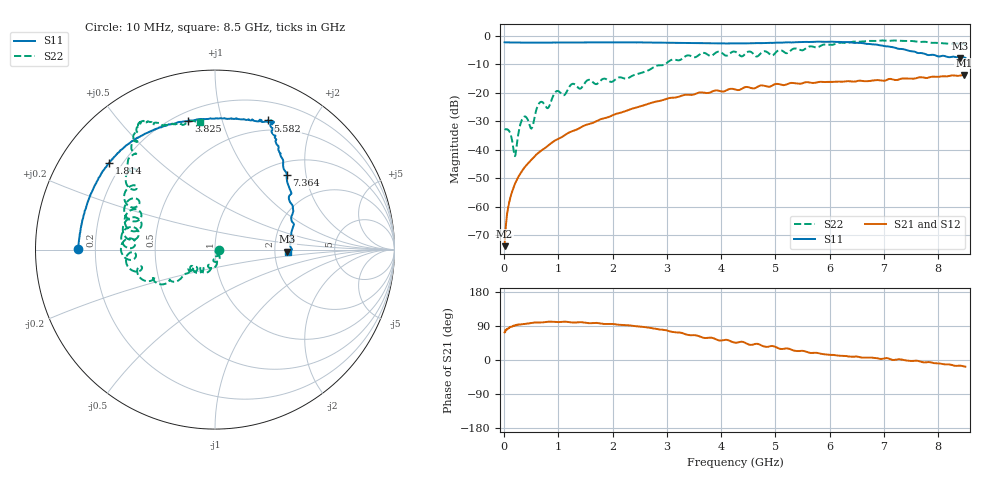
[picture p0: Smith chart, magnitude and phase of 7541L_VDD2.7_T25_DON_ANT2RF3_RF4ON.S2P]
!Agilent Technologies,E5071C,MY46417908,A.11.23
!Date: Wed Dec 09 17:18:27 2020
!Data & Calibration Information:
!Freq	S11:SOLT2(ON)	S21:SOLT2(ON)	S12:SOLT2(ON)	S22:SOLT2(ON)
!PortZ  Port1:50+j0  Port2:50+j0
!Above PortZ is port z conversion or system Z0 setting when saving the data.
!When reading, reference impedance value at option line is always used.
# Hz S dB R 50
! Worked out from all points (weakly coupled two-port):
!   1601 points, 10 MHz to 8.5 GHz, reference 50 ohm
!   highest |S21| = -13.76 dB at 8.468 GHz (marker M1); lowest = -73.8 dB at 10 MHz (marker M2)
!   lowest |S11| = -7.9 dB at 8.41 GHz (marker M3), VSWR 2.35, Z = 117 - j3.32 ohm
!   |S11| at or under -10 dB: nowhere
!   |S22| runs from -42.3 to -1.7 dB; largest |S21 - S12| = 0.0025
!   S11 on the Smith chart (normalised r, x): 10 MHz: 0.13, +0.00; 1.814 GHz: 0.15, +0.35; 3.825 GHz: 0.25, +0.78; 5.582 GHz: 0.39, +1.42; 7.364 GHz: 1.25, +1.56; 8.5 GHz: 2.37, -0.09
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1e7  -2.32 179.6  -73.82 73.0  -73.60 70.5  -32.75 -7.1
8.959375e7  -2.38 177.8  -58.87 84.3  -58.92 85.0  -33.33 -51.8
2.01025e8  -2.39 175.1  -52.02 91.0  -52.02 91.1  -42.26 -46.6
3.336812e8  -2.41 172.1  -47.33 94.3  -47.31 94.7  -29.33 -50.5
5.034812e8  -2.43 168.3  -43.54 97.7  -43.51 97.8  -32.62 -76.4
6.626688e8  -2.43 164.8  -40.65 99.0  -40.66 99.2  -23.36 -79.4
8.059375e8  -2.42 161.5  -38.65 100.9  -38.64 101.0  -25.40 -91.1
9.65125e8  -2.41 157.9  -36.52 100.1  -36.52 100.0  -19.50 -99.6
1.426769e9  -2.37 148.3  -32.03 99.7  -32.03 99.7  -18.30 -121.7
1.814125e9  -2.36 140.5  -29.09 95.5  -29.09 95.5  -15.22 -135.3
2.270462e9  -2.36 131.9  -26.23 92.0  -26.23 92.0  -15.02 -140.8
2.843538e9  -2.45 122.0  -22.98 80.8  -22.99 80.8  -10.41 -145.0
3.825194e9  -2.70 101.7  -19.65 58.7  -19.65 58.7  -7.04 -174.4
4.255e9  -2.75 90.8  -18.84 45.6  -18.84 45.6  -5.62 169.6
4.658275e9  -2.60 80.7  -18.08 42.8  -18.11 42.8  -7.31 162.9
5.581562e9  -2.18 67.7  -16.30 21.1  -16.28 21.2  -4.17 143.2
5.671769e9  -2.19 66.2  -16.56 18.6  -16.51 18.4  -3.77 136.1
7.088538e9  -3.79 55.7  -15.21 3.8  -15.26 3.7  -1.82 120.3
7.364462e9  -4.78 46.2  -15.01 -0.3  -15.01 -0.1  -1.85 118.6
8.409794e9  -7.89 -1.7  -13.92 -15.0  -13.99 -15.0  -2.82 98.8
8.468162e9  -7.60 -1.9  -13.76 -16.7  -13.86 -16.7  -2.93 97.5
8.5e9  -7.78 -2.2  -13.79 -17.6  -13.88 -17.4  -2.92 96.9
